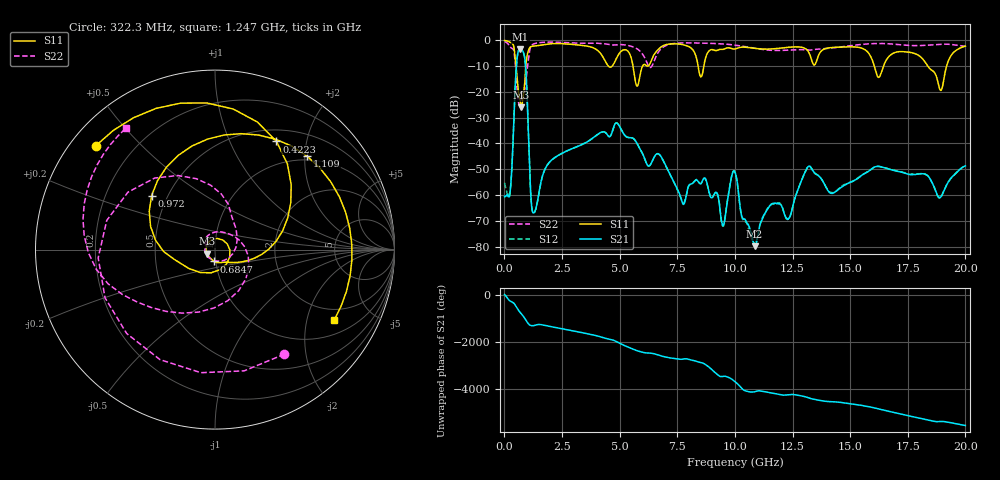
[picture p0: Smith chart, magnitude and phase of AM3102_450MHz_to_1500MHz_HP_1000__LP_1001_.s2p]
!Agilent Technologies,E8364B,MY43040894,A.07.50.67
!Agilent E8364B: A.07.50.67
!Date: Thursday, January 11, 2018 05:58:41
!Correction: S11(Full 2 Port(1,2))
!S21(Full 2 Port(1,2))
!S12(Full 2 Port(1,2))
!S22(Full 2 Port(1,2))
!S2P File: Measurements: S11, S21, S12, S22:
# Hz S  dB  R 50
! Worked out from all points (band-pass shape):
!   1601 points, 10 MHz to 20 GHz, reference 50 ohm
!   highest |S21| = -3.44 dB at 684.7 MHz (marker M1); lowest = -79.8 dB at 10.85 GHz (marker M2)
!   |S21| within 3 dB of the highest: 559.5 MHz to 875.5 MHz (316 MHz wide, 44 % of centre)
!   lowest |S11| = -25.9 dB at 722.1 MHz (marker M3), VSWR 1.11, Z = 45.6 - j2.05 ohm
!   |S11| at or under -10 dB: 504.6 MHz to 929.8 MHz (425.2 MHz wide, 59.3 % of centre); 5.58 GHz to 5.994 GHz (414.5 MHz wide, 7.16 % of centre); 18.37 GHz to 19.18 GHz (817.4 MHz wide, 4.35 % of centre)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
!   |S22| runs from -24.9 to -0.5 dB; largest |S21 - S12| = 0.0016
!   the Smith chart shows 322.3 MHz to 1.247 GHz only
!   S11 on the Smith chart (normalised r, x): 322.3 MHz: 0.07, +0.37; 422.3 MHz: 0.65, +1.51; 684.7 MHz: 0.98, -0.13; 972 MHz: 0.41, +0.31; 1.109 GHz: 0.91, +2.05; 1.247 GHz: 1.54, -2.96
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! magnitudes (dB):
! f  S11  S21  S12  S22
! 10 MHz  -0.1  -60.6  -55.2  -0.5
! 322.3 MHz  -1.1  -50.1  -49.9  -3.1
! 422.3 MHz  -3.2  -28.1  -28.2  -4.7
! 684.7 MHz  -23.6  -3.4  -3.5  -24.9
! 722.1 MHz  -25.9  -3.5  -3.5  -23.8
! 972 MHz  -6.7  -18.8  -18.8  -12.5
! 1.109 GHz  -2.7  -53.4  -53.3  -3.5
! 1.247 GHz  -2.3  -66.9  -66.9  -1.5
! 1.909 GHz  -1.4  -47.8  -47.8  -0.7
! 3.346 GHz  -2.0  -40.5  -40.5  -1.1
! 5.307 GHz  -3.9  -37.5  -37.5  -1.9
! 5.757 GHz  -17.8  -40.0  -40.0  -3.3
! 6.682 GHz  -3.5  -44.0  -44.0  -4.6
! 7.744 GHz  -1.7  -63.5  -63.1  -1.0
! 8.531 GHz  -14.2  -55.6  -55.5  -1.1
! 9.48 GHz  -3.5  -71.9  -72.0  -1.4
! 10.01 GHz  -3.4  -51.1  -51.1  -1.9
! 10.85 GHz  -3.1  -79.8  -79.3  -3.1
! 13.34 GHz  -8.0  -50.0  -49.9  -3.7
! 16.68 GHz  -6.3  -49.9  -49.8  -1.3
! 18.93 GHz  -19.4  -60.8  -60.8  -1.5
! 20 GHz  -2.3  -48.7  -48.7  -2.3
